FUNCTION "Gest Output 2ndCC" : VOID
TITLE =Spia Manuale
VERSION : 0.1

BEGIN
NETWORK
TITLE =Riservato per cassetto controllo corti



//   U     "MG"
//    =     "R160"
NETWORK
TITLE =R 161 = Remote cycle start
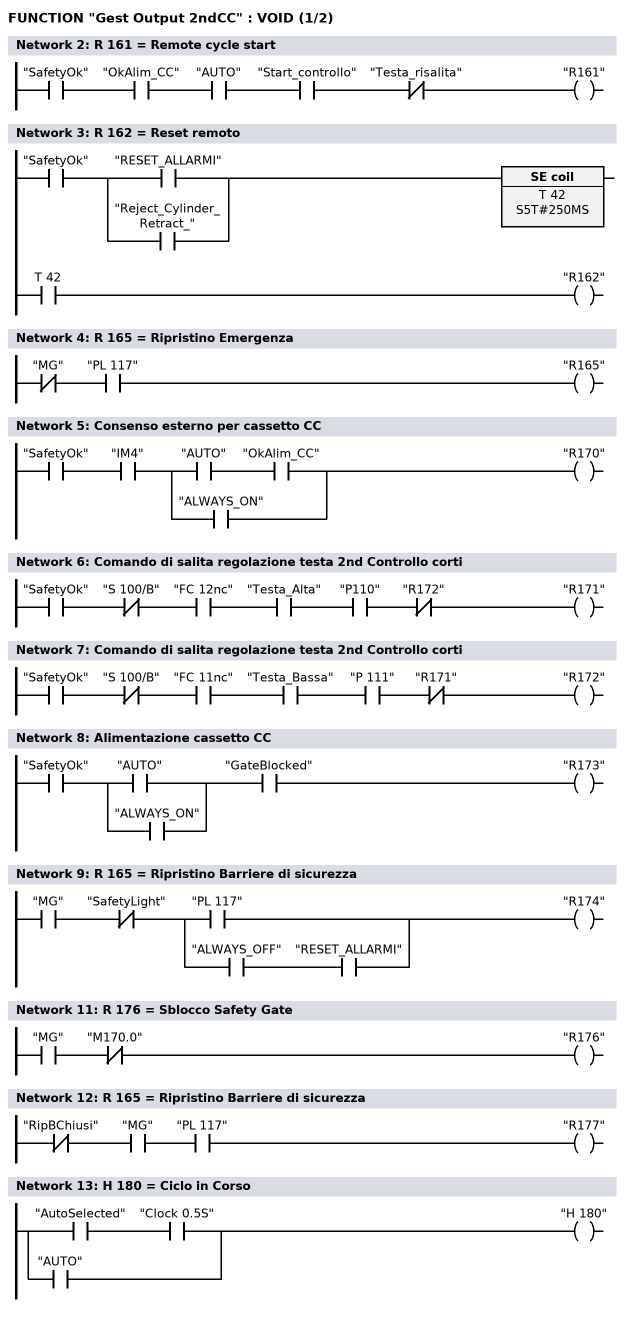
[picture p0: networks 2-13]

      U     "SafetyOk";
      U     "OkAlim_CC";
      U     "AUTO";
      U     "Start_controllo";
      UN    "Testa_risalita";
      =     "R161";
NETWORK
TITLE =R 162 = Reset remoto

      U     "SafetyOk";
      U(    ;
      O     "RESET_ALLARMI";
      O     "Reject_Cylinder_Retract_";
      )     ;
      L     S5T#250MS;
      SV    T     42;
      NOP   0;
      NOP   0;
      NOP   0;
      U     T     42;
      =     "R162";
NETWORK
TITLE =R 165 = Ripristino Emergenza

      UN    "MG";
      U     "PL 117";
      =     "R165";
NETWORK
TITLE =Consenso esterno per cassetto CC

      U     "SafetyOk";
      U     "IM4";
      U(    ;
      U     "AUTO";
      U     "OkAlim_CC";
      O     "ALWAYS_ON";
      )     ;
      =     "R170";
NETWORK
TITLE =Comando di salita regolazione testa 2nd Controllo corti

      U     "SafetyOk";
      UN    "S 100/B";
      U     "FC 12nc";
      U     "Testa_Alta";
      U     "P110";
      UN    "R172";
      =     "R171";
NETWORK
TITLE =Comando di salita regolazione testa 2nd Controllo corti

      U     "SafetyOk";
      UN    "S 100/B";
      U     "FC 11nc";
      U     "Testa_Bassa";
      U     "P 111";
      UN    "R171";
      =     "R172";
NETWORK
TITLE =Alimentazione cassetto CC

      U     "SafetyOk";
      U(    ;
      O     "AUTO";
      O     "ALWAYS_ON";
      )     ;
      U     "GateBlocked";
      =     "R173";
NETWORK
TITLE =R 165 = Ripristino Barriere di sicurezza

      U     "MG";
      UN    "SafetyLight";
      U(    ;
      O     "PL 117";
      O     ;
      U     "ALWAYS_OFF";
      U     "RESET_ALLARMI";
      )     ;
      =     "R174";
NETWORK
TITLE =Riservato R175

NETWORK
TITLE =R 176 = Sblocco Safety Gate

      U     "MG";
      UN    "M170.0";
      =     "R176";
NETWORK
TITLE =R 165 = Ripristino Barriere di sicurezza

      UN    "RipBChiusi";
      U     "MG";
      U     "PL 117";
      =     "R177";
NETWORK
TITLE =H 180 = Ciclo in Corso

      U     "AutoSelected";
      U     "Clock 0.5S";
      O     "AUTO";
      =     "H 180";
NETWORK
TITLE =H 181 = Presenza Allarme
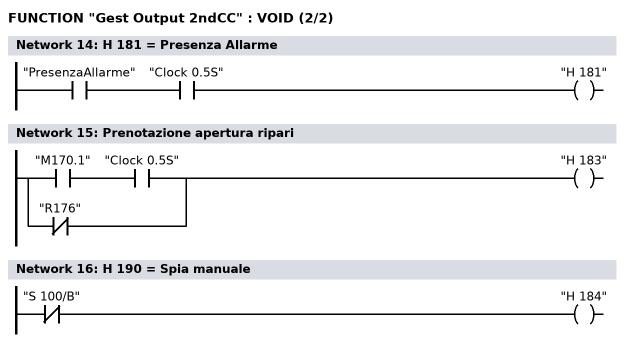
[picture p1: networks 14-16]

      U     "PresenzaAllarme";
      U     "Clock 0.5S";
      =     "H 181";
NETWORK
TITLE =Prenotazione apertura ripari

      U     "M170.1";
      U     "Clock 0.5S";
      ON    "R176";
      =     "H 183";
NETWORK
TITLE =H 190 = Spia manuale

      UN    "S 100/B";
      =     "H 184";
NETWORK
TITLE =Spia di segnalazione scivolo occupato

      U(    ;
      O(    ;
      UN    "Scarico_occupato";
      L     S5T#3S;
      SE    "T44";
      NOP   0;
      NOP   0;
      NOP   0;
      U     "T44";
      )     ;
      O     "H 185";
      )     ;
      UN    "RESET_ALLARMI";
      =     "H 185";
NETWORK
TITLE =Spia segnalazione scarto per DIVE
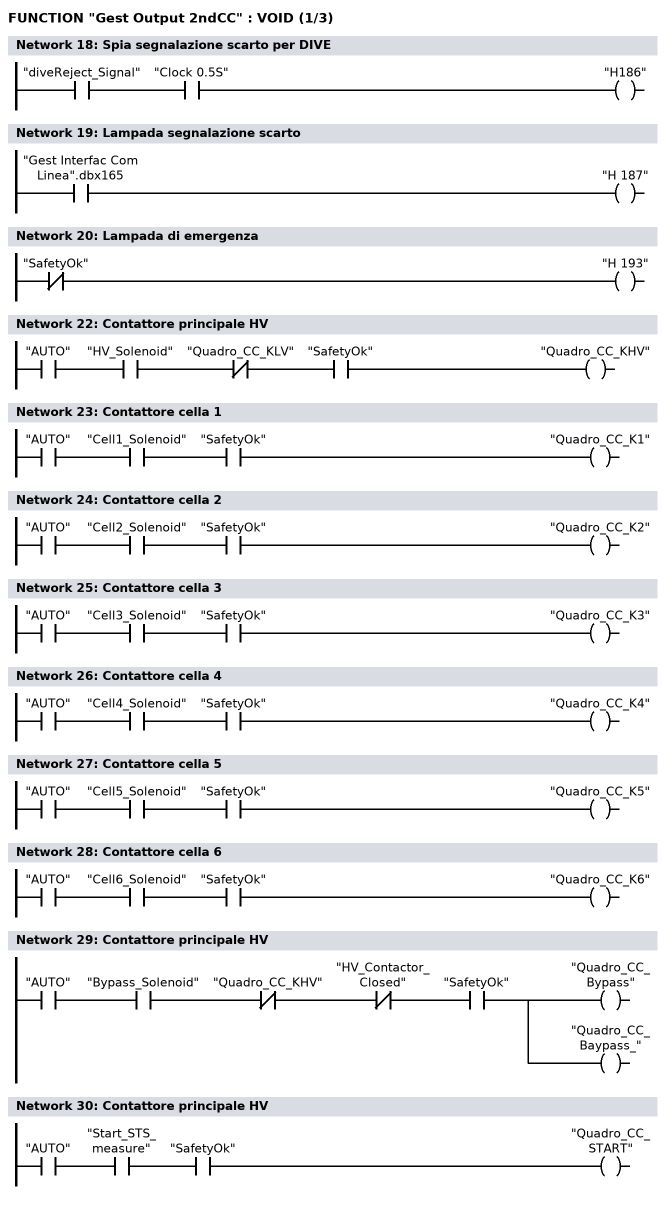
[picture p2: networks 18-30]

      U     "diveReject_Signal";
      U     "Clock 0.5S";
      =     "H186";
NETWORK
TITLE =Lampada segnalazione scarto

      U     "Gest Interfac Com Linea".dbx165;
      =     "H 187";
NETWORK
TITLE =Lampada di emergenza

      UN    "SafetyOk";
      =     "H 193";
NETWORK
TITLE =##################### Inizio gestione STS #################



NETWORK
TITLE =Contattore principale HV

      U     "AUTO";
      U     "HV_Solenoid";
      UN    "Quadro_CC_KLV";
      U     "SafetyOk";
      =     "Quadro_CC_KHV";
NETWORK
TITLE =Contattore cella 1

      U     "AUTO";
      U     "Cell1_Solenoid";
      U     "SafetyOk";
      =     "Quadro_CC_K1";
NETWORK
TITLE =Contattore cella 2

      U     "AUTO";
      U     "Cell2_Solenoid";
      U     "SafetyOk";
      =     "Quadro_CC_K2";
NETWORK
TITLE =Contattore cella 3

      U     "AUTO";
      U     "Cell3_Solenoid";
      U     "SafetyOk";
      =     "Quadro_CC_K3";
NETWORK
TITLE =Contattore cella 4

      U     "AUTO";
      U     "Cell4_Solenoid";
      U     "SafetyOk";
      =     "Quadro_CC_K4";
NETWORK
TITLE =Contattore cella 5

      U     "AUTO";
      U     "Cell5_Solenoid";
      U     "SafetyOk";
      =     "Quadro_CC_K5";
NETWORK
TITLE =Contattore cella 6

      U     "AUTO";
      U     "Cell6_Solenoid";
      U     "SafetyOk";
      =     "Quadro_CC_K6";
NETWORK
TITLE =Contattore principale HV

      U     "AUTO";
      U     "Bypass_Solenoid";
      UN    "Quadro_CC_KHV";
      UN    "HV_Contactor_Closed";
      U     "SafetyOk";
      =     "Quadro_CC_Bypass";
      =     "Quadro_CC_Baypass_";
NETWORK
TITLE =Contattore principale HV

      U     "AUTO";
      U     "Start_STS_measure";
      U     "SafetyOk";
      =     "Quadro_CC_START";
NETWORK
TITLE =Comando discesa testa
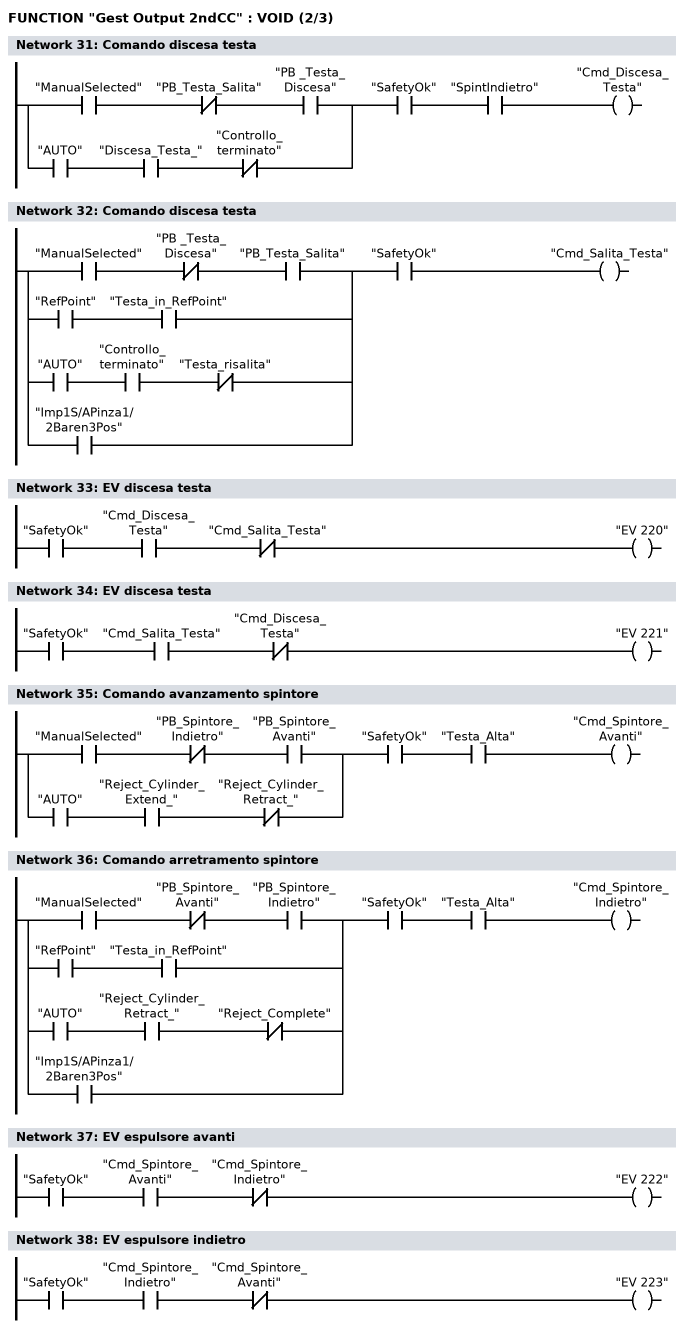
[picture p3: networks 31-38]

      U(    ;
      U     "ManualSelected";
      UN    "PB_Testa_Salita";
      U     "PB _Testa_Discesa";
      O     ;
      U     "AUTO";
      U     "Discesa_Testa_";
      UN    "Controllo_terminato";
      )     ;
      U     "SafetyOk";
      U     "SpintIndietro";
      =     "Cmd_Discesa_Testa";
NETWORK
TITLE =Comando discesa testa

      U(    ;
      U     "ManualSelected";
      UN    "PB _Testa_Discesa";
      U     "PB_Testa_Salita";
      O     ;
      U     "RefPoint";
      U     "Testa_in_RefPoint";
      O     ;
      U     "AUTO";
      U     "Controllo_terminato";
      UN    "Testa_risalita";
      O     "Imp1S/APinza1/2Baren3Pos";
      )     ;
      U     "SafetyOk";
      =     "Cmd_Salita_Testa";
NETWORK
TITLE =EV discesa testa

      U     "SafetyOk";
      U     "Cmd_Discesa_Testa";
      UN    "Cmd_Salita_Testa";
      =     "EV 220";
NETWORK
TITLE =EV discesa testa

      U     "SafetyOk";
      U     "Cmd_Salita_Testa";
      UN    "Cmd_Discesa_Testa";
      =     "EV 221";
NETWORK
TITLE =Comando avanzamento spintore

      U(    ;
      U     "ManualSelected";
      UN    "PB_Spintore_Indietro";
      U     "PB_Spintore_Avanti";
      O     ;
      U     "AUTO";
      U     "Reject_Cylinder_Extend_";
      UN    "Reject_Cylinder_Retract_";
      )     ;
      U     "SafetyOk";
      U     "Testa_Alta";
      =     "Cmd_Spintore_Avanti";
NETWORK
TITLE =Comando arretramento spintore

      U(    ;
      U     "ManualSelected";
      UN    "PB_Spintore_Avanti";
      U     "PB_Spintore_Indietro";
      O     ;
      U     "RefPoint";
      U     "Testa_in_RefPoint";
      O     ;
      U     "AUTO";
      U     "Reject_Cylinder_Retract_";
      UN    "Reject_Complete";
      O     "Imp1S/APinza1/2Baren3Pos";
      )     ;
      U     "SafetyOk";
      U     "Testa_Alta";
      =     "Cmd_Spintore_Indietro";
NETWORK
TITLE =EV espulsore avanti

      U     "SafetyOk";
      U     "Cmd_Spintore_Avanti";
      UN    "Cmd_Spintore_Indietro";
      =     "EV 222";
NETWORK
TITLE =EV espulsore indietro

      U     "SafetyOk";
      U     "Cmd_Spintore_Indietro";
      UN    "Cmd_Spintore_Avanti";
      =     "EV 223";
NETWORK
TITLE =H 250 = Spia di Ref Point
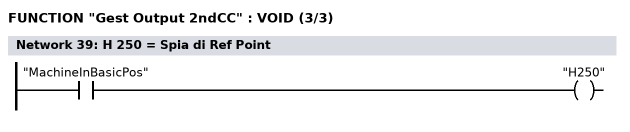
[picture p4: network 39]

      U     "MachineInBasicPos";
      =     "H250";
END_FUNCTION

